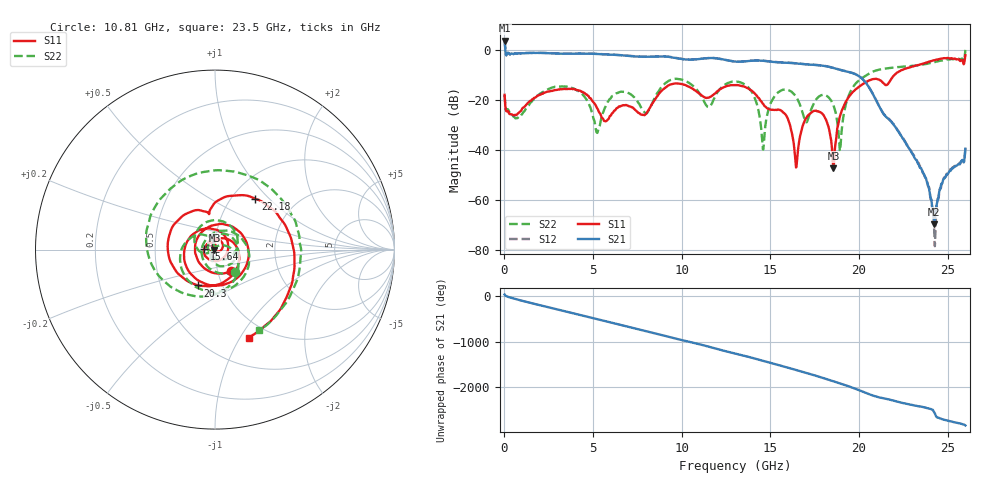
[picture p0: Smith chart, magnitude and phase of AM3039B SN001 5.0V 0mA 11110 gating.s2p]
!Agilent Technologies,E8364B,MY43040894,A.07.50.67
!Agilent E8364B: A.07.50.67
!Date: Tuesday, June 28, 2016 08:13:16
!Correction: S11(Full 2 Port(1,2))
!S21(Full 2 Port(1,2))
!S12(Full 2 Port(1,2))
!S22(Full 2 Port(1,2))
!S2P File: Measurements: S11, S21, S12, S22:
# Hz S  dB  R 50
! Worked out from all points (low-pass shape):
!   1601 points, 10 MHz to 26 GHz, reference 50 ohm
!   highest |S21| = 3.91 dB at 10 MHz (marker M1); lowest = -69.8 dB at 24.25 GHz (marker M2)
!   |S21| within 3 dB of the highest: start of sweep to 43.88 MHz
!   lowest |S11| = -47.4 dB at 18.56 GHz (marker M3), VSWR 1.01, Z = 49.7 - j0.259 ohm
!   |S11| at or under -10 dB: start of sweep to 21.99 GHz
!   |S22| runs from -40.4 to 0.2 dB; largest |S21 - S12| = 0.023
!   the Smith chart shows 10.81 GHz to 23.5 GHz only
!   S11 on the Smith chart (normalised r, x): 10.81 GHz: 1.16, -0.29; 15.64 GHz: 0.89, +0.01; 20.3 GHz: 0.77, -0.32; 22.18 GHz: 1.28, +0.83; 23.5 GHz: 0.80, -1.09
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1e7  -17.85 53.7  3.91 41.1  3.96 41.8  -17.90 22.3
7.734562e8  -25.29 37.2  -1.23 -73.9  -1.18 -73.7  -26.91 -4.7
1.796812e9  -18.62 -41.0  -1.02 -174.9  -0.97 -174.7  -18.57 -62.5
2.885144e9  -15.94 -172.2  -1.26 81.5  -1.21 81.7  -14.66 175.2
4.347081e9  -16.65 8.7  -1.31 -55.9  -1.28 -55.8  -17.37 5.4
5.516631e9  -27.16 -90.8  -1.57 -169.3  -1.51 -169.1  -25.84 0.4
6.539988e9  -22.52 -125.9  -1.95 91.6  -1.89 91.7  -16.65 -105.4
7.5471e9  -25.08 98.3  -2.52 -4.5  -2.47 -4.4  -21.07 117.5
8.684162e9  -17.76 -125.9  -2.45 -113.4  -2.38 -113.2  -16.56 -132.6
1.081209e10  -16.42 -53.0  -3.62 41.4  -3.57 41.3  -15.46 -47.8
1.3005e10  -13.91 -76.9  -4.50 179.2  -4.46 178.9  -12.52 -94.6
1.458064e10  -21.42 37.4  -4.20 17.6  -4.16 17.3  -39.76 145.5
1.563649e10  -24.28 175.7  -4.88 -95.0  -4.83 -95.1  -16.03 112.1
1.646492e10  -46.83 -44.3  -5.26 173.5  -5.21 173.3  -18.77 -5.0
1.734208e10  -24.77 120.0  -5.77 74.5  -5.74 74.3  -22.99 101.2
1.856036e10  -47.41 -142.3  -7.11 -75.3  -7.06 -75.3  -22.10 -90.9
2.029844e10  -13.12 -115.1  -12.25 42.6  -12.23 42.7  -10.53 -123.8
2.167916e10  -13.04 97.2  -27.61 -114.3  -27.49 -113.7  -7.15 93.1
2.218272e10  -8.84 51.4  -32.24 -166.9  -32.07 -166.7  -6.71 47.2
2.349846e10  -5.58 -69.1  -47.26 86.1  -47.11 83.2  -5.82 -61.1
2.424568e10  -4.00 -132.0  -69.85 -40.7  -73.37 -37.5  -4.77 -118.8
2.6e10  -1.94 33.2  -39.48 30.3  -39.10 29.8  0.19 64.3
